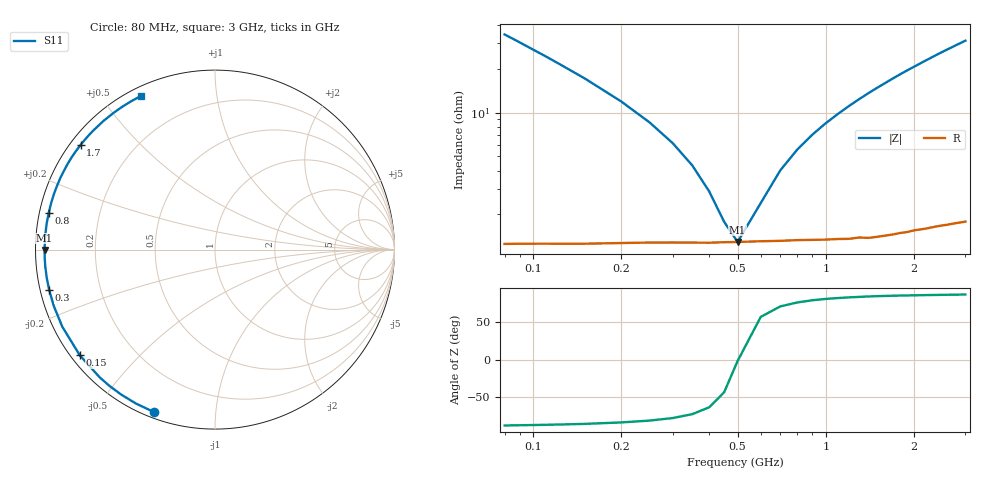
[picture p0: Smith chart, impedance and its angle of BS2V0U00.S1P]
! SIEMENS Small Signal Semiconductors
! BB640
! Si Tuning Diode in SOD323
! VR = 2 V
! S-Parameters:  July  1993
# GHz  S  MA  R  50
!  f  S11
! GHz  MAG  ANG
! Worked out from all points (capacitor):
!   33 points, 80 MHz to 3 GHz, reference 50 ohm
!   read as one part to ground: C = 56.1 pF near 80 MHz
!   lowest |Z| = 1.29 ohm at 500 MHz (marker M1)
!   series resonance near 502.1 MHz, so ESL is about 1.8 nH
!   S11 on the Smith chart (normalised r, x): 80 MHz: 0.03, -0.69; 150 MHz: 0.03, -0.34; 300 MHz: 0.03, -0.12; 800 MHz: 0.03, +0.11; 1.7 GHz: 0.03, +0.34; 3 GHz: 0.04, +0.63
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0.08  0.9667 -110.7
0.09  0.9641 -117.2
0.1  0.962 -122.9
0.11  0.9603 -127.7
0.12  0.959 -132.0
0.15  0.9561 -142.0
0.2  0.9531 -153.2
0.25  0.9515 -160.7
0.3  0.9508 -166.2
0.35  0.9505 -170.5
0.4  0.9504 -174.1
0.45  0.9499 -177.2
0.5  0.9497 -179.9
0.6  0.9492 175.4
0.7  0.9491 171.3
0.8  0.9488 167.6
0.9  0.949 164.2
1  0.9492 161.0
1.2  0.9496 155.1
1.4  0.95 149.6
1.6  0.9495 144.5
1.7  0.9493 142.0
2  0.9484 135.1
2.2  0.9486 130.8
2.4  0.9485 126.7
2.6  0.949 122.9
2.8  0.9494 119.3
3  0.9501 115.9
